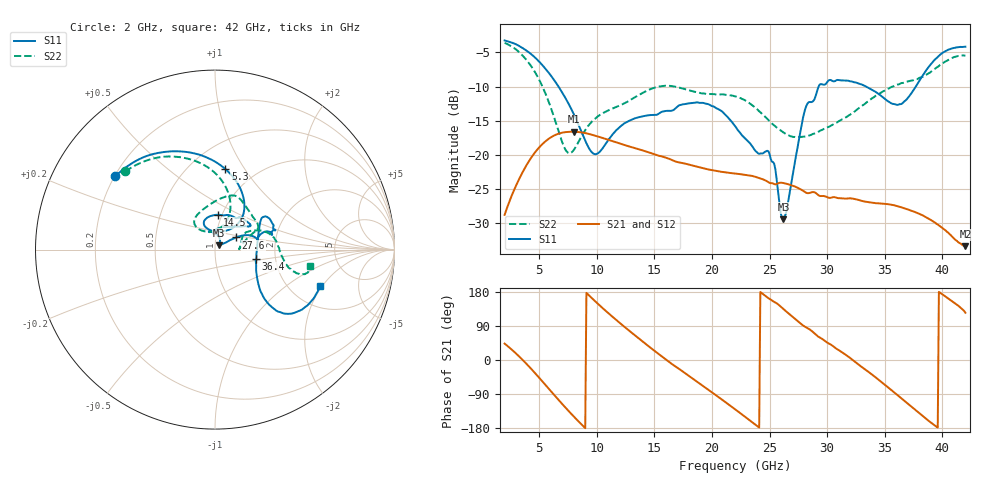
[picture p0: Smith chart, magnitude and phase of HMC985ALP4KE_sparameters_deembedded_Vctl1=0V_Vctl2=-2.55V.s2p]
!s2p File: Measurements: S11, S21, S12, S22
# GHz S dB R 50.0
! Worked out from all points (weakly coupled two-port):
!   401 points, 2 GHz to 42 GHz, reference 50 ohm
!   highest |S21| = -16.64 dB at 8 GHz (marker M1); lowest = -33.4 dB at 42 GHz (marker M2)
!   lowest |S11| = -29.5 dB at 26.2 GHz (marker M3), VSWR 1.07, Z = 52.3 + j2.55 ohm
!   |S11| at or under -10 dB: 6.677 GHz to 29.26 GHz (22.59 GHz wide, 126 % of centre); 33.37 GHz to 37.7 GHz (4.323 GHz wide, 12.2 % of centre)
!   |S22| runs from -19.8 to -3.6 dB; largest |S21 - S12| = 0.00062
!   S11 on the Smith chart (normalised r, x): 2 GHz: 0.20, +0.32; 5.3 GHz: 0.73, +0.82; 14.5 GHz: 0.95, +0.38; 27.6 GHz: 1.25, +0.17; 36.4 GHz: 1.58, -0.18; 42 GHz: 2.91, -1.90
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2  -3.23 143.6  -28.85 43.2  -28.84 43.2  -3.58 138.9
3.5  -4.28 116.9  -22.79 2.3  -22.80 2.2  -5.35 108.8
5.3  -6.90 82.6  -18.42 -57.2  -18.44 -57.2  -10.05 75.7
7.2  -11.45 52.9  -16.72 -122.9  -16.74 -122.9  -18.99 82.4
8  -14.04 48.6  -16.64 -149.0  -16.63 -149.0  -19.32 112.8
8.7  -16.77 52.6  -16.74 -170.8  -16.74 -170.8  -17.24 127.0
10  -19.89 89.4  -17.29 151.0  -17.28 151.1  -14.50 128.0
14.5  -14.22 85.8  -19.66 36.3  -19.64 36.3  -10.51 79.5
15.4  -13.96 73.6  -20.17 15.3  -20.18 15.2  -10.00 72.7
19.3  -12.42 34.0  -22.02 -70.1  -22.01 -70.1  -11.00 43.4
22  -15.79 52.3  -22.78 -129.8  -22.81 -129.9  -11.44 26.5
25  -19.93 99.0  -24.15 161.3  -24.12 161.3  -15.09 16.6
26.2  -29.50 46.5  -24.17 134.6  -24.22 134.5  -16.74 6.6
27.6  -17.32 29.9  -25.00 98.6  -25.01 98.5  -17.40 1.1
28.1  -13.27 21.0  -25.53 87.4  -25.58 87.3  -17.33 2.6
28.7  -12.25 13.0  -25.51 75.6  -25.51 75.6  -17.01 6.6
31  -9.05 23.3  -26.40 26.2  -26.38 26.1  -15.10 27.2
33.3  -9.93 34.2  -26.91 -24.9  -26.89 -25.0  -12.51 26.4
35.4  -12.27 12.0  -27.31 -75.0  -27.29 -75.1  -10.24 17.7
36.4  -12.58 -13.2  -27.71 -100.3  -27.75 -100.3  -9.52 11.9
39.5  -5.82 -43.4  -30.18 -176.1  -30.10 -176.0  -7.20 -14.4
42  -4.15 -18.9  -33.44 124.7  -33.46 124.3  -5.42 -9.9
